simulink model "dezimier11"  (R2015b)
settings: Solver=VariableStepAuto  StartTime=0.0  StopTime=10.0  RelTol=1e-3
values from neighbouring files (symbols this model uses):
  a = 1/(Tsig/2.5)    (= 7.8125)    [fourier_transf_puls_3.m]    (also in fourier_transf_puls_4.m; schar_1.m = 5)
  b = 10    [schar_1.m]
  M = 5    [dezimier_1.m]    (also in dezimier_11.m; dezimier_2.m; dezimier_3.m; farrow_3.m)
  Ts = 1/fs    (= 5e-05)    [basisband_1.m]    (also in basisband_2.m = 5e-06; dezimier_1.m = 0.0005; dezimier_11.m = 0.0005; dezimier_2.m = 0.0005)
libraries: dspsigops x1

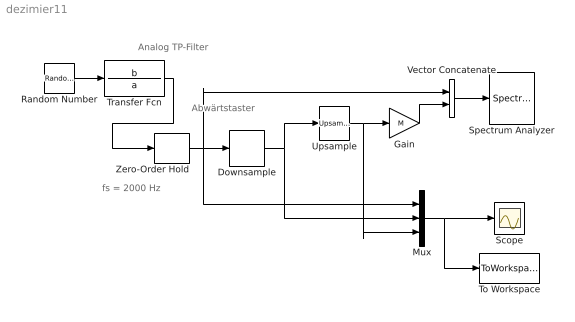
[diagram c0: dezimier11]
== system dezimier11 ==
  note: Abwärtstaster
  note: fs = 2000 Hz
  note: Analog TP-Filter
  Downsample : DownSample  N=M  RateOptions=Allow multirate processing
  Gain : Gain  Gain=M
  Mux : Mux  Inputs=3
  Random Number : RandomNumber  Seed=25678  SampleTime=Ts/10
  Scope : Scope
  Spectrum Analyzer : SpectrumAnalyzer
  To Workspace : ToWorkspace  VariableName=y  SaveFormat=Timeseries  SampleTime=-1
  Transfer Fcn : TransferFcn  Numerator=b  Denominator=a
  Upsample : dspsigops/Upsample  N=M  phase=0  RateOptions=Allow multirate processing  ic=0  mode=Unused parameter value
  Vector Concatenate : Concatenate  Mode=Multidimensional array  ConcatenateDimension=2
  Zero-Order Hold : ZeroOrderHold  SampleTime=Ts
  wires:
  Random Number/1 -> Transfer Fcn/1
  Transfer Fcn/1 -> Zero-Order Hold/1
  Mux/1 -> To Workspace/1, Scope/1
  Zero-Order Hold/1 -> Vector Concatenate/1, Mux/1, Downsample/1
  Downsample/1 -> Mux/2, Upsample/1
  Upsample/1 -> Mux/3, Gain/1
  Vector Concatenate/1 -> Spectrum Analyzer/1
  Gain/1 -> Vector Concatenate/2
